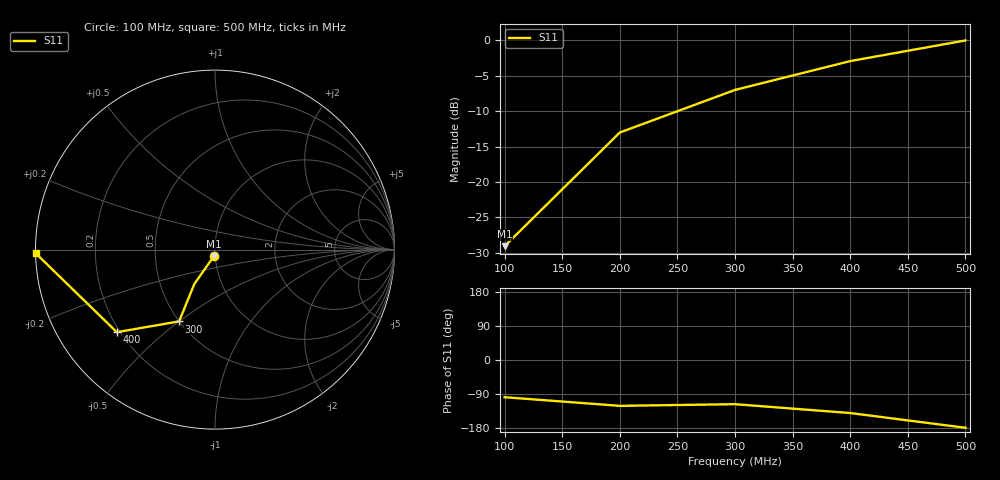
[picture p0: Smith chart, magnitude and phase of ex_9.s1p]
!1-port Z-parameter file, multiple frequency points
# MHz Z MA R 75
!freq magZ11 angZ11
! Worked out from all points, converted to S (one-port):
!   5 points, 100 MHz to 500 MHz, reference 75 ohm
!   lowest |S11| = -29.0 dB at 100 MHz (marker M1), VSWR 1.07, Z = 74.1 - j5.18 ohm
!   |S11| at or under -10 dB: start of sweep to 249.9 MHz
!   S11 on the Smith chart (normalised r, x): 100 MHz: 0.99, -0.07; 300 MHz: 0.50, -0.50; 400 MHz: 0.19, -0.35; 500 MHz: 0.00, -0.01
100  0.99 -4.0
200  0.8 -22.0
300  0.707 -45.0
400  0.4 -62.0
500  0.01 -89.0
